|   This file is an IBIS representation of the   |
|   Integrated Device Technology Inc   |
|   IDT8V89316   |
|   Ethernet PLL for Industrial Automation and Power Systems   |
[IBIS Ver]   4.1
[File name]   8v89316.ibs
[File Rev]   1.1
|Rev 1.1,  Apr 14, 2014
|Created separate RLC package for non-Power signals
|Rev 1.0, 28 May 2013
|Original Model
[Notes]
The RLC values, including the power pins, have a max of >35pF capacitance. Some
simulators may use this value for a Min corner simulation of output signals, which
leads to incorrect results.  A separate Component was created to include only the
non-Power RLC values for these cases.  Use "IDT8V89316-NonPowerRLC-BGA" to simulate
switching signals.
[Date]   14 Apr 2014
[Source]   Originated at Integrated Device Technology, Inc.
[Disclaimer]
IDT hereby grants the user of this IBIS model a non-exclusive,
nontransferable license to use this IBIS model under the following terms.
Before using this IBIS model, the user should read this license.
If the user does not accept these terms,  the IBIS model should be
returned to IDT within 30 days.
   The user is granted this license only to use the IBIS model and
is not granted rights to sell, load, rent, lease or license the IBIS
model in whole or in part, or in modified form to anyone other than
user. User may modify the IBIS model to suit its specific
applications but rights to derivative works and such modifications
shall belong to IDT.
   This IBIS model is provided on an AS IS basis and IDT makes
absolutely no warranty with respect to the information contained
herein. IDT DISCLAIMS AND CUSTOMER WAIVES ALL WARRANTIES, EXPRESS
OR IMPLIED, INCLUDING WARRANTIES OF MERCHANTABILITY OR FITNESS FOR
A PARTICULAR PURPOSE. The entire risk as to quality and performance
is with the Customer. ACCORDINGLY, IN NO EVENT SHALL THE COMPANY BE
LIABLE FOR ANY DAMAGES, WHETHER IN CONTRACT OR TORT,INCLUDING ANY
LOST PROFITS OR OTHER INCIDENTAL, CONSEQUENTIAL, EXEMPLARY, OR
PUNITIVE DAMAGES ARISING OUT OF THE USE OR APPLICATION OF THE IBIS
model provided in this package. Further, IDT reserves the right to
make changes without notice to any product herein to improve
reliability, function, or design. IDT does not convey any license
under patent rights or any other intellectual property rights,
including those of third parties.
   IDT is not obligated to provide maintenance or support
for the licensed IBIS model.
[Copyright]   Copyright 2013 by IDT Inc.
[Component]   IDT8V89316-NonPowerRLC-BGA
[Manufacturer] Integrated Device Technology, Inc.
[Package]
|BGA 196
|lead + wire   typ   min   max
R_pkg   0.222   0.0515674   0.628939
L_pkg   3.206nH   0.886nH   9.061nH
C_pkg   1.171pF   0.497pF   3.985pF
[Pin]   signal_name   model_name   R_pin   L_pin   C_pin
A1   NC   NC   0.334348   4.73633nH   1.50284pF
A2   VDDA0   POWER   0.08402   1.24995nH   4.93195pF
A3   OUT6_NEG   SG_OPECL07_100H   0.340484   5.61005nH   1.29913pF
A4   NC   NC
A5   NC   NC
A6   IC1   NC
A7   IC1   NC
A8   TDI   PDUSDGZ   0.142959   2.16014nH   0.622557pF
A9   VC0   NC
A10   IC2   NC
A11   OSCI   NC
A12   TMS   PDUSDGZ   0.158506   2.27988nH   0.666767pF
A13   VC4   NC
A14   TRST   PDDSDGZ   0.164723   2.1921nH   0.675437pF
B1   NC   NC
B2   VSSA0   GND
B3   OUT6_POS   SG_OPECL07_100H   0.278229   4.23554nH   1.78426pF
B4   VSSA   GND
B5   NC   NC
B6   IC1   NC
B7   IC1   NC
B8   TDO   PDT02DGZ   0.176917   2.41141nH   0.655527pF
B9   VSSA0   GND
B10   TCK   PDDSDGZ   0.221025   2.95269nH   0.841653pF
B11   VSSA   GND
B12   VSSA   GND
B13   VSSD0   GND
B14   VDDD0   POWER   0.0371692   0.689269nH   5.71412pF
C1   NC   NC
C2   VDDA0   POWER   0.08402   1.24995nH   4.93195pF
C3   NC   NC
C4   NC   NC
C5   IC1   NC
C6   IC1   NC
C7   VDDDO   POWER   0.0515674   0.886249nH   3.58412pF
C8   VSSDO   GND
C9   VDDA   POWER   0.0753102   1.19036nH   3.15432pF
C10   VSSA   GND
C11   VDDA   POWER   0.0753102   1.19036nH   3.15432pF
C12   VDDA   POWER   0.08402   1.24995nH   4.93195pF
C13   INT_REQ   PDT02DGZ   0.133505   1.88864nH   0.636295pF
C14   IC1   NC
D1   VSSA0   GND
D2   VSSA0   GND
D3   NC   NC
D4   VSSA0   GND
D5   VDDA0   POWER   0.0753102   1.19036nH   3.15432pF
D6   IC1   NC
D7   VSSD   GND
D8   VDDD   POWER   0.0733794   1.32964nH   1.20295pF
D9   IC1   NC
D10   VDDA   POWER   0.0753102   1.19036nH   3.15432pF
D11   VSSA   GND
D12   VDDA   POWER   0.0753102   1.19036nH   3.15432pF
D13   IC1   NC
D14   IC1   NC
E1   OUT5_NEG   SG_OPECL07_100H   0.334819   4.75366nH   1.5807pF
E2   OUT5_POS   SG_OPECL07_100H   0.284387   4.11262nH   1.33295pF
E3   VSSA   GND
E4   VSSA0   GND
E5   VSSA0   GND
E6   IC3   NC
E7   VSSD   GND
E8   VDDD   POWER   0.0733794   1.32964nH   1.20295pF
E9   IC1   NC
E10   VSSA   GND
E11   VDDA   POWER   0.0753102   1.19036nH   3.15432pF
E12   VSSA   GND
E13   IC1   NC
E14   IC1   NC
F1   VDDA0   POWER   0.0186506   0.320268nH   17.9991pF
F2   VSSA0   GND
F3   VSSA0   GND
F4   VSSA0   GND
F5   VDDA0   POWER   0.0753102   1.19036nH   3.15432pF
F6   VSSA0   GND
F7   VSSD   GND
F8   VDDD   POWER   0.0733794   1.32964nH   1.20295pF
F9   VSSD   GND
F10   VDDD   POWER   0.0733794   1.32964nH   1.20295pF
F11   IC1   NC
F12   VDDDO   POWER   0.094203   1.48743nH   2.89182pF
F13   OUT7   PDO04CDG   0.155809   2.11446nH   0.660969pF
F14   VSSDO   GND
G1   VSSA0   GND
G2   VDDA0   POWER   0.0276409   0.422404nH   35.2531pF
G3   VSSA0   GND
G4   VSSA0   GND
G5   VSSA0   GND
G6   VSSD   GND
G7   VDDD   POWER   0.068222   0.90552nH   5.32678pF
G8   IC1   NC
G9   VDDD   POWER   0.0371692   0.689269nH   5.71412pF
G10   VSSD   GND
G11   IC1   GND
G12   IC1   GND
G13   IC1   GND
G14   IC1   GND
H1   VDDA0   POWER   0.068222   0.90552nH   5.32678pF
H2   VSSA0   GND
H3   VDDAO   POWER   0.08402   1.24995nH   4.93195pF
H4   VSSA0   GND
H5   VSSAO   GND
H6   VSSAO   GND
H7   VSSD   GND
H8   VDDD   POWER   0.068222   0.90552nH   5.32678pF
H9   VSSD   GND
H10   VDDD   POWER   0.068222   0.90552nH   5.32678pF
H11   IC1   NC
H12   IC1   NC
H13   RST   PDUSDGZ   0.83377   12.1862nH   3.88243pF
H14   IN1   ami_rx   0.196725   2.76061nH   0.726838pF
J1   OUT4_NEG   SG_OPECL07_100H   0.252954   3.53133nH   0.730914pF
J2   OUT4_POS   SG_OPECL07_100H   0.246367   3.34809nH   0.699321pF
J3   VDDAO   POWER   0.08402   1.24995nH   4.93195pF
J4   VSSAO   GND
J5   VDDAO   POWER   0.08402   1.24995nH   4.93195pF
J6   VSSAO   GND
J7   VDDAO   POWER   0.08402   1.24995nH   4.93195pF
J8   VSSAO   GND
J9   VSSA   GND
J10   VDDA   POWER   0.0753102   1.19036nH   3.15432pF
J11   DPLL_LOCK   PDT02DGZ   0.131397   2.24181nH   0.729437pF
J12   IC1   NC
J13   IN2   ami_rx   0.160825   2.31934nH   0.67745pF
J14   IN3   ami_rx   0.362282   5.2171nH   1.60392pF
K1   VSSAO   GND
K2   VSSAO   GND
K3   VSSAO   GND
K4   VDDAO   POWER   0.08402   1.24995nH   4.93195pF
K5   VSSAO   GND
K6   VDDAO   POWER   0.08402   1.24995nH   4.93195pF
K7   VSSAO   GND
K8   VSSD   GND
K9   VDDD   POWER   0.068222   0.90552nH   5.32678pF
K10   VSSAO   GND
K11   IC1   NC
K12   IC1   NC
K13   I2C_SCL   PDDSDGZ   0.601196   9.0618nH   2.89322pF
K14   I2C_SDA   PDD02SDGZ   0.283464   4.89492nH   3.98528pF
L1   OUT3_NEG   SG_OPECL07_100H   0.172003   2.36707nH   0.531051pF
L2   OUT3_POS   SG_OPECL07_100H   0.158041   2.1493nH   0.497244pF
L3   VDDA0   POWER   0.08402   1.24995nH   4.93195pF
L4   VSSAO   GND
L5   VSSAO   GND
L6   VSSAO   GND
L7   VSSAO   GND
L8   I2C_AD1   PDUSDGZ   0.628939   7.3282nH   3.17476pF
L9   I2C_AD2   PDUSDGZ   0.579908   7.18207nH   2.82964pF
L10   CAP1   NC
L11   VSSA   GND
L12   CAP2   NC
L13   VSSA   GND
L14   CAP3   NC
M1   VDDAO   POWER   0.08402   1.24995nH   4.93195pF
M2   VSSAO   GND
M3   VSSAO   GND
M4   VSSADO   GND
M5   VDDAO   POWER   0.08402   1.24995nH   4.93195pF
M6   VSSAO   GND
M7   VDDAO   POWER   0.08402   1.24995nH   4.93195pF
M8   VSSAO   GND
M9   VSSAO   GND
M10   VSSAO   GND
M11   VSSAO   GND
M12   NC   NC
M13   NC   NC
M14   NC   NC
N1   VSSAO   GND
N2   OUT2_POS   SG_OPECL07_100H   0.134275   1.83601nH   0.60374pF
N3   VSSAO   GND
N4   OUT1_POS   PECL_LVDS04   0.134275   1.83601nH   0.60374pF
N5   VSSAO   GND
N6   IN_APLL2_POS INDIFF01P_PDPU100K   0.264444   3.49073nH   0.768733pF
N7   IC2   NC
N8   I2C   NC
N9   VSSA   GND
N10   XTAL_OUT   NC   0.180966   2.37539nH   0.741578pF
N11   VSSA   GND
N12   APLL1_LF1   NC   0.159345   2.18796nH   1.07785pF
N13   VSSAO   GND
N14   VSSA   GND
P1   VDDAO   POWER   0.08402   1.24995nH   4.93195pF
P2   OUT2_NEG   SG_OPECL07_100H   0.226993   3.03703nH   0.665671pF
P3   VSSAO   GND
P4   OUT1_NEG   PECL_LVDS04   0.226993   3.03703nH   0.665671pF
P5   VDDAO   POWER   0.068222   0.90552nH   5.32678pF
P6   IN_APLL_NEG  INDIFF01N_PDPU100K   0.340484   5.61005nH   1.29913pF
P7   IC2   NC
P8   IC2   NC
P9   VDDA   POWER   0.0753102   1.19036nH   3.15432pF
P10   XTAL_IN   NC   0.163448   2.22776nH   0.674849pF
P11   VDDA   POWER   0.08402   1.24995nH   4.93195pF
P12   APLL_LFO   NC   0.214835   2.96596nH   1.55911pF
P13   ISET_APLL   NC   0.256779   3.60749nH   1.80531pF
P14   VDDA   POWER   0.0753102   1.19036nH   3.15432pF
[Diff Pin]   inv_pin vdiff   tdelay_typ   tdelay_min   tdelay_max
|Inputs
N6   P6   150mV   NA   NA   NA
|Outputs
N4   P4   NA   0   0   0
N2   P2   NA   0   0   0
L2   L1   NA   0   0   0
J2   J1   NA   0   0   0
E2   E1   NA   0   0   0
B3   A3   NA   0   0   0
[Component]   IDT8V89316-BGA-POWER-RLC
[Manufacturer] Integrated Device Technology, Inc.
[Package]
|BGA 196
|lead + wire   typ   min   max
R_pkg   0.3069   0.01865   1.0645
L_pkg   4.3859nF   0.32027nF   16.561nF
C_pkg   2.7933pF   0.49724pF   35.307pF
[Pin]   signal_name   model_name   R_pin   L_pin   C_pin
A1   NC   NC   0.334348   4.73633nH   1.50284pF
A2   VDDA0   POWER   0.08402   1.24995nH   4.93195pF
A3   OUT6_NEG   SG_OPECL07_100H   0.340484   5.61005nH   1.29913pF
A4   NC   NC
A5   NC   NC
A6   IC1   NC
A7   IC1   NC
A8   TDI   PDUSDGZ   0.142959   2.16014nH   0.622557pF
A9   VC0   NC
A10   IC2   NC
A11   OSCI   NC
A12   TMS   PDUSDGZ   0.158506   2.27988nH   0.666767pF
A13   VC4   NC
A14   TRST   PDDSDGZ   0.164723   2.1921nH   0.675437pF
B1   NC   NC
B2   VSSA0   GND
B3   OUT6_POS   SG_OPECL07_100H   0.278229   4.23554nH   1.78426pF
B4   VSSA   GND
B5   NC   NC
B6   IC1   NC
B7   IC1   NC
B8   TDO   PDT02DGZ   0.176917   2.41141nH   0.655527pF
B9   VSSA0   GND
B10   TCK   PDDSDGZ   0.221025   2.95269nH   0.841653pF
B11   VSSA   GND
B12   VSSA   GND
B13   VSSD0   GND
B14   VDDD0   POWER   0.0371692   0.689269nH   5.71412pF
C1   NC   NC
C2   VDDA0   POWER   0.08402   1.24995nH   4.93195pF
C3   NC   NC
C4   NC   NC
C5   IC1   NC
C6   IC1   NC
C7   VDDDO   POWER   0.0515674   0.886249nH   3.58412pF
C8   VSSDO   GND
C9   VDDA   POWER   0.0753102   1.19036nH   3.15432pF
C10   VSSA   GND
C11   VDDA   POWER   0.0753102   1.19036nH   3.15432pF
C12   VDDA   POWER   0.08402   1.24995nH   4.93195pF
C13   INT_REQ   PDT02DGZ   0.133505   1.88864nH   0.636295pF
C14   IC1   NC
D1   VSSA0   GND
D2   VSSA0   GND
D3   NC   NC
D4   VSSA0   GND
D5   VDDA0   POWER   0.0753102   1.19036nH   3.15432pF
D6   IC1   NC
D7   VSSD   GND
D8   VDDD   POWER   0.0733794   1.32964nH   1.20295pF
D9   IC1   NC
D10   VDDA   POWER   0.0753102   1.19036nH   3.15432pF
D11   VSSA   GND
D12   VDDA   POWER   0.0753102   1.19036nH   3.15432pF
D13   IC1   NC
D14   IC1   NC
E1   OUT5_NEG   SG_OPECL07_100H   0.334819   4.75366nH   1.5807pF
E2   OUT5_POS   SG_OPECL07_100H   0.284387   4.11262nH   1.33295pF
E3   VSSA   GND
E4   VSSA0   GND
E5   VSSA0   GND
E6   IC3   NC
E7   VSSD   GND
E8   VDDD   POWER   0.0733794   1.32964nH   1.20295pF
E9   IC1   NC
E10   VSSA   GND
E11   VDDA   POWER   0.0753102   1.19036nH   3.15432pF
E12   VSSA   GND
E13   IC1   NC
E14   IC1   NC
F1   VDDA0   POWER   0.0186506   0.320268nH   17.9991pF
F2   VSSA0   GND
F3   VSSA0   GND
F4   VSSA0   GND
F5   VDDA0   POWER   0.0753102   1.19036nH   3.15432pF
F6   VSSA0   GND
F7   VSSD   GND
F8   VDDD   POWER   0.0733794   1.32964nH   1.20295pF
F9   VSSD   GND
F10   VDDD   POWER   0.0733794   1.32964nH   1.20295pF
F11   IC1   NC
F12   VDDDO   POWER   0.094203   1.48743nH   2.89182pF
F13   OUT7   PDO04CDG   0.155809   2.11446nH   0.660969pF
F14   VSSDO   GND
G1   VSSA0   GND
G2   VDDA0   POWER   0.0276409   0.422404nH   35.2531pF
G3   VSSA0   GND
G4   VSSA0   GND
G5   VSSA0   GND
G6   VSSD   GND
G7   VDDD   POWER   0.068222   0.90552nH   5.32678pF
G8   IC1   NC
G9   VDDD   POWER   0.0371692   0.689269nH   5.71412pF
G10   VSSD   GND
G11   IC1   GND
G12   IC1   GND
G13   IC1   GND
G14   IC1   GND
H1   VDDA0   POWER   0.068222   0.90552nH   5.32678pF
H2   VSSA0   GND
H3   VDDAO   POWER   0.08402   1.24995nH   4.93195pF
H4   VSSA0   GND
H5   VSSAO   GND
H6   VSSAO   GND
H7   VSSD   GND
H8   VDDD   POWER   0.068222   0.90552nH   5.32678pF
H9   VSSD   GND
H10   VDDD   POWER   0.068222   0.90552nH   5.32678pF
H11   IC1   NC
H12   IC1   NC
H13   RST   PDUSDGZ   0.83377   12.1862nH   3.88243pF
H14   IN1   ami_rx   0.196725   2.76061nH   0.726838pF
J1   OUT4_NEG   SG_OPECL07_100H   0.252954   3.53133nH   0.730914pF
J2   OUT4_POS   SG_OPECL07_100H   0.246367   3.34809nH   0.699321pF
J3   VDDAO   POWER   0.08402   1.24995nH   4.93195pF
J4   VSSAO   GND
J5   VDDAO   POWER   0.08402   1.24995nH   4.93195pF
J6   VSSAO   GND
J7   VDDAO   POWER   0.08402   1.24995nH   4.93195pF
J8   VSSAO   GND
J9   VSSA   GND
J10   VDDA   POWER   0.0753102   1.19036nH   3.15432pF
J11   DPLL_LOCK   PDT02DGZ   0.131397   2.24181nH   0.729437pF
J12   IC1   NC
J13   IN2   ami_rx   0.160825   2.31934nH   0.67745pF
J14   IN3   ami_rx   0.362282   5.2171nH   1.60392pF
K1   VSSAO   GND
K2   VSSAO   GND
K3   VSSAO   GND
K4   VDDAO   POWER   0.08402   1.24995nH   4.93195pF
K5   VSSAO   GND
K6   VDDAO   POWER   0.08402   1.24995nH   4.93195pF
K7   VSSAO   GND
K8   VSSD   GND
K9   VDDD   POWER   0.068222   0.90552nH   5.32678pF
K10   VSSAO   GND
K11   IC1   NC
K12   IC1   NC
K13   I2C_SCL   PDDSDGZ   0.601196   9.0618nH   2.89322pF
K14   I2C_SDA   PDD02SDGZ   0.283464   4.89492nH   3.98528pF
L1   OUT3_NEG   SG_OPECL07_100H   0.172003   2.36707nH   0.531051pF
L2   OUT3_POS   SG_OPECL07_100H   0.158041   2.1493nH   0.497244pF
L3   VDDA0   POWER   0.08402   1.24995nH   4.93195pF
L4   VSSAO   GND
L5   VSSAO   GND
L6   VSSAO   GND
L7   VSSAO   GND
L8   I2C_AD1   PDUSDGZ   0.628939   7.3282nH   3.17476pF
L9   I2C_AD2   PDUSDGZ   0.579908   7.18207nH   2.82964pF
L10   CAP1   NC
L11   VSSA   GND
L12   CAP2   NC
L13   VSSA   GND
L14   CAP3   NC
M1   VDDAO   POWER   0.08402   1.24995nH   4.93195pF
M2   VSSAO   GND
M3   VSSAO   GND
M4   VSSADO   GND
M5   VDDAO   POWER   0.08402   1.24995nH   4.93195pF
M6   VSSAO   GND
M7   VDDAO   POWER   0.08402   1.24995nH   4.93195pF
M8   VSSAO   GND
M9   VSSAO   GND
M10   VSSAO   GND
M11   VSSAO   GND
M12   NC   NC
M13   NC   NC
M14   NC   NC
N1   VSSAO   GND
N2   OUT2_POS   SG_OPECL07_100H   0.134275   1.83601nH   0.60374pF
N3   VSSAO   GND
N4   OUT1_POS   PECL_LVDS04   0.134275   1.83601nH   0.60374pF
N5   VSSAO   GND
N6   IN_APLL2_POS INDIFF01P_PDPU100K   0.264444   3.49073nH   0.768733pF
N7   IC2   NC
N8   I2C   NC
N9   VSSA   GND
N10   XTAL_OUT   NC   0.180966   2.37539nH   0.741578pF
N11   VSSA   GND
N12   APLL1_LF1   NC   0.159345   2.18796nH   1.07785pF
N13   VSSAO   GND
N14   VSSA   GND
P1   VDDAO   POWER   0.08402   1.24995nH   4.93195pF
P2   OUT2_NEG   SG_OPECL07_100H   0.226993   3.03703nH   0.665671pF
P3   VSSAO   GND
P4   OUT1_NEG   PECL_LVDS04   0.226993   3.03703nH   0.665671pF
P5   VDDAO   POWER   0.068222   0.90552nH   5.32678pF
P6   IN_APLL_NEG  INDIFF01N_PDPU100K   0.340484   5.61005nH   1.29913pF
P7   IC2   NC
P8   IC2   NC
P9   VDDA   POWER   0.0753102   1.19036nH   3.15432pF
P10   XTAL_IN   NC   0.163448   2.22776nH   0.674849pF
P11   VDDA   POWER   0.08402   1.24995nH   4.93195pF
P12   APLL_LFO   NC   0.214835   2.96596nH   1.55911pF
P13   ISET_APLL   NC   0.256779   3.60749nH   1.80531pF
P14   VDDA   POWER   0.0753102   1.19036nH   3.15432pF
[Diff Pin]   inv_pin vdiff   tdelay_typ   tdelay_min   tdelay_max
|Inputs
N6   P6   150mV   NA   NA   NA
|Outputs
N4   P4   NA   0   0   0
N2   P2   NA   0   0   0
L2   L1   NA   0   0   0
J2   J1   NA   0   0   0
E2   E1   NA   0   0   0
B3   A3   NA   0   0   0
| Models and submodels in the file (10): PECL_LVDS04 (Output_ECL), PDDSDGZ (Input), PDUSDGZ (Input), ami_rx (Input), PDT02DGZ (3-state), PDD02SDGZ (I/O), PDO04CDG (Output), INDIFF01P_PDPU100K (Input), INDIFF01N_PDPU100K (Input), SG_OPECL07_100H (Output_ECL)
